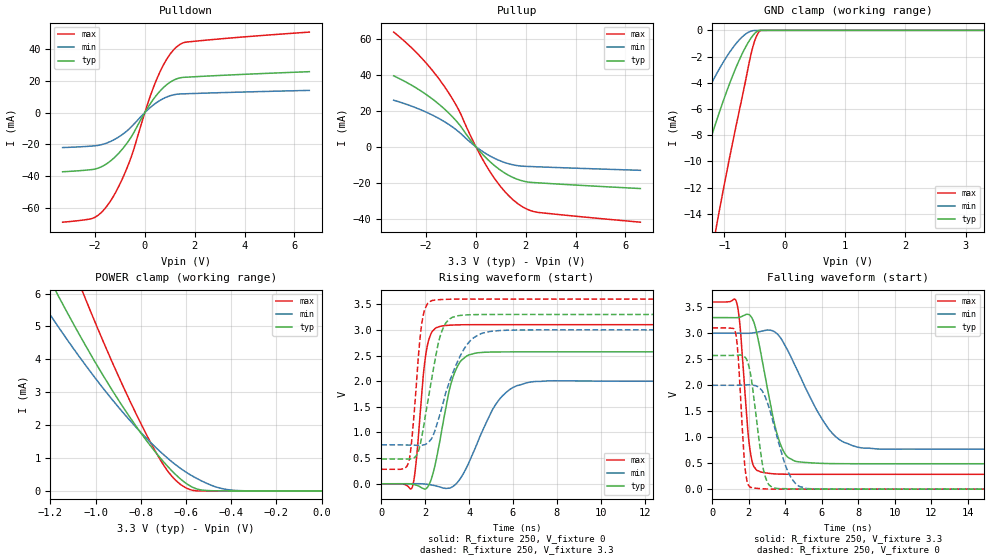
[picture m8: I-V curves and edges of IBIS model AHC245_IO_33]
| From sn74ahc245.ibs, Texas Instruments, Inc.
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[Model]   AHC245_IO_33
Model_type  I/O
Vinl = 0.9
Vinh = 2.1
Enable   Active-Low
|Vref =   0.0
|Rref =   1000
Cref =   50p
Vmeas =   1.65
| variable   typ   min   max
C_comp   2.54pF   2.40pF   2.63pF
| C_pullup   3.38pF   2.65pF   3.86pF
| C_pulldown   3.61pF   2.55pF   4.85pF
| C_tri-state   2.54pF   2.40pF   2.63pF
[Temperature Range]   40   100   -40
| Ambient temperature   25   85   -40
[Voltage range]   3.3   3   3.6
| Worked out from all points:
|   slope of the pulldown table from 0 to 0.495 V, typ, clamps not added: 43.2 ohm
|   slope of the pullup table from 0 to 0.495 V, typ, clamps not added: 67 ohm
|   GND clamp passes 1 mA (typ) near -0.61 V on its own axis
|   POWER clamp passes 1 mA (typ) near -0.71 V on its own axis
|   rising waveform, R_fixture 250, V_fixture 0: 20-80 % time 725ps typ, 1.32ns min, 384ps max; typ from 0.001 V to 2.57 V
|   falling waveform, R_fixture 250, V_fixture 3.3: 20-80 % time 966ps typ, 1.97ns min, 430ps max; typ from 3.3 V to 0.488 V
|   rising waveform, R_fixture 250, V_fixture 3.3: 20-80 % time 696ps typ, 1.1ns min, 380ps max; typ from 0.484 V to 3.3 V
|   falling waveform, R_fixture 250, V_fixture 0: 20-80 % time 562ps typ, 992ps min, 312ps max; typ from 2.57 V to 0.001 V
[GND Clamp]
| AHC245_IO_33
|   Voltage   I(typ)   I(min)   I(max)
-3.3V     -45.05mA   -27.92mA   -79.88mA
-2.245V   -25.21mA   -14.96mA   -46.47mA
-2.195V   -24.31mA   -14.37mA   -44.95mA
-1.64V    -14.72mA   -8.194mA   -28.59mA
-1.375V   -10.49mA   -5.527mA   -21.27mA
-1.135V   -6.957mA   -3.36mA    -15.03mA
-1.1V     -6.472mA   -3.07mA    -14.15mA
-845mV    -3.251mA   -1.232mA   -8.143mA
-590mV    -808uA     -118.9uA   -2.472mA
-485mV    -175.7uA   -11.58uA   -633.5uA
-390mV    -186.6nA   -4.991uA   -3.664uA
3.3V      54.37pA    1.353uA    45pA
[POWER Clamp]
| AHC245_IO_33
|   Voltage   I(typ)   I(min)   I(max)
-3.3V     44.21mA    34.59mA    61.32mA
-1.255V   7.137mA    5.922mA    9.636mA
-1.165V   5.936mA    4.993mA    7.959mA
-1.045V   4.43mA     3.83mA     5.848mA
-925mV    3.049mA    2.766mA    3.896mA
-780mV    1.58mA     1.638mA    1.783mA
-695mV    853.3uA    1.078mA    744.4uA
-630mV    397.8uA    714.9uA    228.8uA
-595mV    208.6uA    549.3uA    76.59uA
-545mV    45.57uA    353.3uA    17.81nA
-430mV    794.3nA    55.84uA    137.5pA
-48.03fV  54.37pA    187.8pA    59.5pA
[Pulldown]
| AHC245_IO_33
|   Voltage   I(typ)   I(min)   I(max)
-3.3V     -37.2mA    -21.99mA   -68.91mA
-2.055V   -35.67mA   -20.95mA   -66.2mA
-1.72V    -33.87mA   -20.08mA   -62.37mA
-1.375V   -30.36mA   -18.13mA   -55.5mA
-995mV    -24.64mA   -14.79mA   -44.74mA
-615mV    -16.93mA   -10.07mA   -30.77mA
130mV     3.398mA    1.959mA    6.36mA
515mV     11.84mA    6.735mA    22.38mA
920mV     18.05mA    10.06mA    34.59mA
1.325V    21.47mA    11.61mA    41.95mA
1.67V     22.25mA    11.85mA    44.33mA
6.6V      25.72mA    13.95mA    50.6mA
[Pullup]
| AHC245_IO_33
|   Voltage   I(typ)   I(min)   I(max)
-3.3V     39.41mA    25.86mA    63.72mA
-2.275V   31.61mA    20.9mA     50.72mA
-1.81V    27.19mA    18.03mA    43.48mA
-1.385V   22.48mA    14.92mA    35.87mA
-715mV    13.14mA    8.594mA    21.16mA
-30mV     500.9uA    317uA      824.1uA
510mV     -7.582mA   -4.704mA   -12.64mA
1.075V    -13.89mA   -8.388mA   -23.56mA
1.635V    -17.94mA   -10.44mA   -31.15mA
2.05V     -19.53mA   -10.94mA   -34.69mA
2.46V     -20.05mA   -11.16mA   -36.45mA
6.6V      -23.26mA   -13.12mA   -41.95mA
[Ramp]
| AHC245_IO_33
| variable   typ   min   max
dV/dt_r   1.61/7.91E-10   1.26/1.43E-09   1.92/4.07E-10
dV/dt_f   1.73/1.02E-09   1.38/2.05E-09   2.02/4.59E-10
R_load = 250
[Rising Waveform]
| AHC245_IO_33
R_fixture =   250
C_fixture =   0
L_fixture =   0
V_fixture =   0
V_fixture_min = 0
V_fixture_max = 0
|   Time   V(typ)   V(min)   V(max)
0s        700.2uV    1.113mV    387.2uV
1.405ns   -6.335mV   1.693mV    -72.48mV
1.575ns   -24.07mV   2.376mV    377.3mV
2.09ns    -75.29mV   -10.01mV   2.675V
2.825ns   1.212V     -83.46mV   3.079V
3.28ns    2.097V     -47.19mV   3.094V
3.835ns   2.472V     273.1mV    3.1V
5.345ns   2.57V      1.626V     3.101V
6.935ns   2.571V     1.991V     3.101V
49.99ns   2.571V     1.998V     3.1V
[Falling Waveform]
| AHC245_IO_33
R_fixture =   250
C_fixture =   0
L_fixture =   0
V_fixture =   3.3
V_fixture_min = 3
V_fixture_max = 3.6
|   Time   V(typ)   V(min)   V(max)
0s        3.299V     2.999V     3.6V
1.33ns    3.298V     2.999V     3.59V
1.52ns    3.31V      2.998V     3.127V
2.085ns   3.335V     3V         706.4mV
2.8ns     2.35V      3.046V     320.6mV
3.49ns    1.137V     3.006V     292.3mV
4.11ns    623mV      2.683V     287mV
6.44ns    492mV      1.129V     285.6mV
8.165ns   488.6mV    794.4mV    285.7mV
49.99ns   488.2mV    767.4mV    285.5mV
[Rising Waveform]
| AHC245_IO_33
R_fixture =   250
C_fixture =   0
L_fixture =   0
V_fixture =   3.3
V_fixture_min = 3
V_fixture_max = 3.6
|   Time   V(typ)   V(min)   V(max)
0s        484.1mV    759.4mV    283.6mV
1.25ns    483.9mV    755.4mV    426.5mV
1.415ns   491.2mV    753.5mV    974.5mV
1.845ns   920.1mV    752.1mV    3.123V
2.34ns    2.155V     923.1mV    3.574V
2.66ns    2.842V     1.337V     3.589V
3.01ns    3.169V     1.868V     3.596V
3.95ns    3.293V     2.736V     3.6V
5.09ns    3.3V       2.976V     3.6V
49.99ns   3.299V     2.999V     3.6V
[Falling Waveform]
| AHC245_IO_33
R_fixture =   250
C_fixture =   0
L_fixture =   0
V_fixture =   0
V_fixture_min = 0
V_fixture_max = 0
|   Time   V(typ)   V(min)   V(max)
0s        2.571V     1.998V     3.1V
1.26ns    2.573V     1.998V     3.021V
1.415ns   2.578V     1.998V     2.546V
1.8ns     2.535V     2.003V     382.7mV
2.215ns   1.927V     2V         23.26mV
2.725ns   516.6mV    1.894V     8.449mV
3.04ns    117.7mV    1.639V     2.937mV
4.165ns   7.612mV    323.7mV    -5.161uV
5.2ns     808.2uV    10.72mV    -73.91uV
49.99ns   682.5uV    1.152mV    390.2uV
